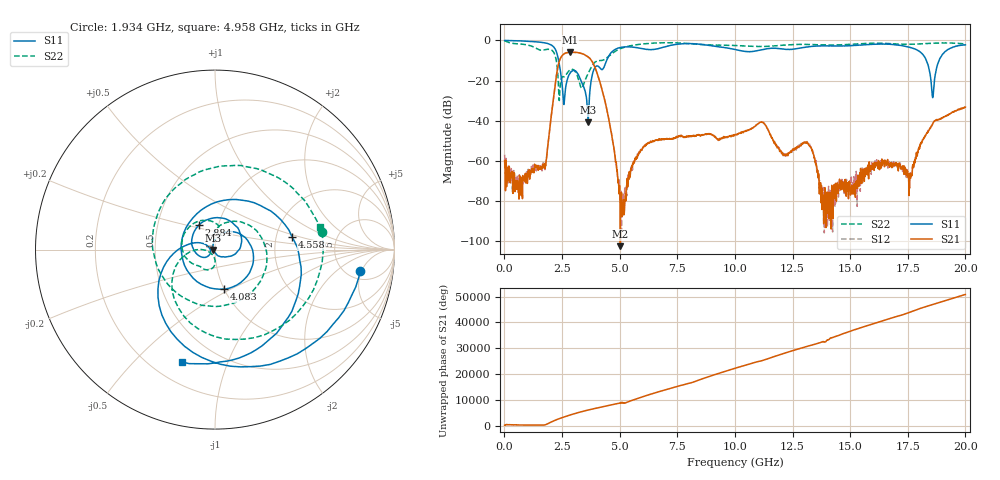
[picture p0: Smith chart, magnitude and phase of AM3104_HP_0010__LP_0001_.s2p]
!Created with skrf (http://scikit-rf.org).
# Hz S RI R 50.0
!freq ReS11 ImS11 ReS21 ImS21 ReS12 ImS12 ReS22 ImS22
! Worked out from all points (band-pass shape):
!   1601 points, 10 MHz to 20 GHz, reference 50 ohm
!   highest |S21| = -5.85 dB at 2.846 GHz (marker M1); lowest = -102.4 dB at 5.032 GHz (marker M2)
!   |S21| within 3 dB of the highest: 2.434 GHz to 3.702 GHz (1.268 GHz wide, 41.3 % of centre)
!   lowest |S11| = -40.7 dB at 3.633 GHz (marker M3), VSWR 1.02, Z = 49.1 - j0.209 ohm
!   |S11| at or under -10 dB: 2.353 GHz to 4.435 GHz (2.083 GHz wide, 61.4 % of centre); 18.31 GHz to 18.85 GHz (547.4 MHz wide, 2.95 % of centre)
!   |S22| runs from -29.9 to -0.2 dB; largest |S21 - S12| = 0.0047
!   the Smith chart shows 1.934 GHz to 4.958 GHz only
!   S11 on the Smith chart (normalised r, x): 1.934 GHz: 6.64, -4.70; 2.884 GHz: 0.81, +0.23; 4.083 GHz: 1.00, -0.46; 4.558 GHz: 2.45, +0.43; 4.958 GHz: 0.32, -0.70
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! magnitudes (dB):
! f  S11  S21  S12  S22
! 10 MHz  0.0  -59.7  -56.8  -0.2
! 759.6 MHz  -0.2  -68.0  -73.2  -1.8
! 1.709 GHz  -1.1  -63.2  -62.9  -4.8
! 1.934 GHz  -1.7  -47.5  -47.5  -4.4
! 2.359 GHz  -10.4  -11.3  -11.3  -25.8
! 2.584 GHz  -31.9  -6.7  -6.7  -18.1
! 2.846 GHz  -16.3  -5.8  -5.9  -14.7
! 2.884 GHz  -15.7  -5.9  -5.9  -14.4
! 3.346 GHz  -20.7  -6.5  -6.5  -23.8
! 3.633 GHz  -40.7  -8.2  -8.2  -16.4
! 4.083 GHz  -12.9  -18.4  -18.4  -10.1
! 4.558 GHz  -7.2  -41.0  -40.9  -7.6
! 4.958 GHz  -3.7  -72.2  -70.6  -4.5
! 5.032 GHz  -3.5  -102.4  -80.7  -4.1
! 6.682 GHz  -4.1  -49.6  -49.2  -1.2
! 10.01 GHz  -4.5  -47.0  -47.0  -2.5
! 13.34 GHz  -2.9  -54.5  -54.7  -2.1
! 13.95 GHz  -2.7  -93.1  -84.5  -2.2
! 16.68 GHz  -1.8  -62.0  -60.9  -1.5
! 17.6 GHz  -3.5  -67.6  -66.0  -1.9
! 18.59 GHz  -28.4  -41.4  -41.4  -1.4
! 20 GHz  -2.2  -33.2  -33.1  -1.7
